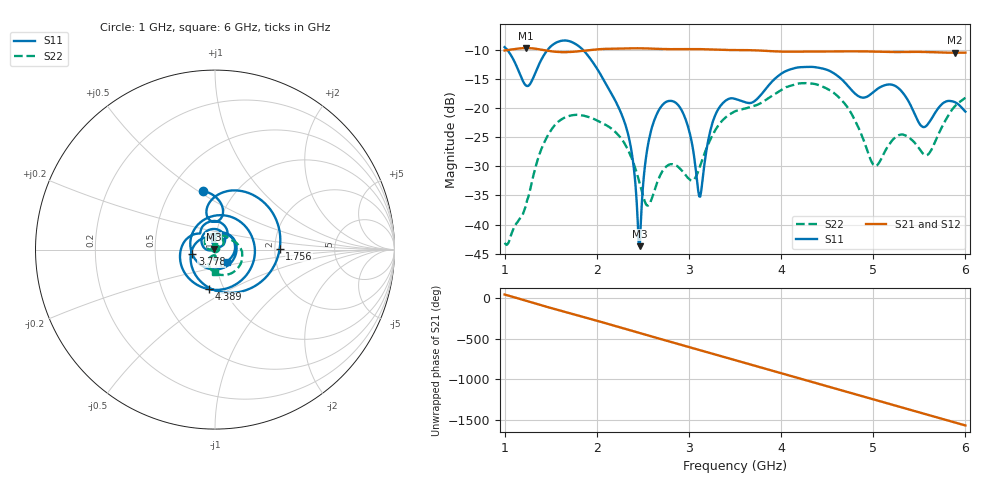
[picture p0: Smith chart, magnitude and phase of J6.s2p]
!Agilent Technologies,E8364B,MY43040528,A.07.50.67
!Agilent E8364B: A.07.50.67
!Date: Sunday, March 01, 2026 18:26:18
!Correction: S11(Full 2 Port(1,2))
!S21(Full 2 Port(1,2))
!S12(Full 2 Port(1,2))
!S22(Full 2 Port(1,2))
!S2P File: Measurements: S11, S21, S12, S22:
# Hz S  dB  R 50
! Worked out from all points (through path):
!   451 points, 1 GHz to 6 GHz, reference 50 ohm
!   highest |S21| = -9.69 dB at 1.233 GHz (marker M1); lowest = -10.5 dB at 5.889 GHz (marker M2)
!   group delay of S21, straight-line fit = 897 ps
!   lowest |S11| = -43.7 dB at 2.467 GHz (marker M3), VSWR 1.01, Z = 49.4 + j0.274 ohm
!   |S11| at or under -10 dB: 1.028 GHz to 1.466 GHz (438.1 MHz wide, 35.1 % of centre); 1.85 GHz to end of sweep
!   |S22| runs from -43.5 to -15.7 dB; largest |S21 - S12| = 0.0014
!   S11 on the Smith chart (normalised r, x): 1 GHz: 0.71, +0.52; 1.756 GHz: 2.13, +0.03; 3.778 GHz: 0.77, -0.04; 4.389 GHz: 0.85, -0.40; 6 GHz: 1.13, -0.15
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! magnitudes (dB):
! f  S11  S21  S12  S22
! 1 GHz  -9.5  -10.1  -10.1  -43.1
! 1.233 GHz  -16.1  -9.7  -9.7  -36.7
! 1.467 GHz  -10.0  -10.2  -10.2  -24.7
! 1.756 GHz  -8.9  -10.3  -10.3  -21.2
! 1.844 GHz  -9.9  -10.2  -10.2  -21.3
! 2.311 GHz  -22.9  -9.8  -9.8  -26.3
! 2.467 GHz  -43.7  -9.7  -9.8  -33.0
! 2.544 GHz  -27.4  -9.8  -9.8  -36.7
! 2.667 GHz  -20.5  -9.8  -9.9  -32.3
! 2.922 GHz  -20.4  -9.9  -9.9  -30.7
! 3.122 GHz  -35.2  -9.9  -9.9  -29.9
! 3.278 GHz  -21.5  -10.0  -10.0  -24.0
! 3.5 GHz  -18.4  -10.0  -10.1  -20.6
! 3.778 GHz  -17.8  -10.1  -10.1  -19.2
! 4.344 GHz  -12.9  -10.3  -10.3  -15.8
! 4.389 GHz  -13.0  -10.3  -10.3  -15.9
! 4.711 GHz  -15.9  -10.2  -10.3  -19.6
! 5.011 GHz  -17.1  -10.3  -10.3  -29.9
! 5.167 GHz  -15.9  -10.4  -10.4  -26.4
! 5.544 GHz  -23.3  -10.4  -10.4  -27.9
! 5.889 GHz  -19.0  -10.5  -10.5  -19.6
! 6 GHz  -20.6  -10.5  -10.5  -18.2
